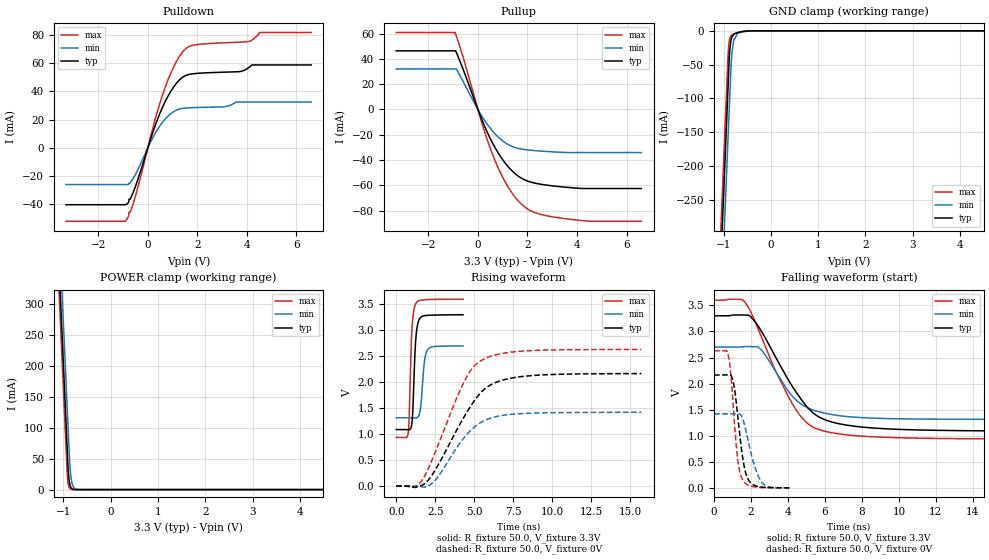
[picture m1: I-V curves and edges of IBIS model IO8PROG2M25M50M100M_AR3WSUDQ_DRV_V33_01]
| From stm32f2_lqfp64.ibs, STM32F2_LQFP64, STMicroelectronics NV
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| *** New cell (Generated with 5.14beta1 (Sep 20 2010 13:23:23))
[Model]   IO8PROG2M25M50M100M_AR3WSUDQ_DRV_V33_01
Model_type 3-state
Polarity   Non-Inverting
Enable   Active-Low
| CAP_THRESHOLD on pad IOV33 is "CMOS" :
| Rising=10.0% of vddio   Falling=90.0% of vddio
| C_comp min and max val. don't necessarily correlate with the min and max pvt
| but are the smallest and greatest pad capacitance found.
| var   typ   min   max
C_comp   2.51830pF  2.40455pF  2.66130pF
Vmeas = 1.65V   | Reference voltage for timing measurements
Cref  = 50.0pF   | Timing specification test load capacitance value
Rref  = 1.0MOhm   | Timing specification test load resistance value
Vref  = 1.65V   | Timing specification test load voltage
[Model Spec]
| variable   typ   min   max
[Temperature Range] 25.0 125.0 -40.0
| variable   typ   min   max
[Voltage Range] 3.3V 2.7V 3.6V
| variable   typ   min   max
[POWER Clamp Reference] 3.3V 2.7V 3.6V
| variable   typ   min   max
[GND Clamp Reference] 0V 0V 0V
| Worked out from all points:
|   slope of the pulldown table from 0 to 0.495 V, typ, clamps not added: 20 ohm
|   slope of the pullup table from 0 to 0.495 V, typ, clamps not added: 21.7 ohm
|   GND clamp passes 1 mA (typ) near -0.59 V on its own axis
|   POWER clamp passes 1 mA (typ) near -0.81 V on its own axis
|   rising waveform, R_fixture 50.0, V_fixture 3.3V: 20-80 % time 186ps typ, 225ps min, 175ps max; typ from 1.09 V to 3.3 V
|   falling waveform, R_fixture 50.0, V_fixture 3.3V: 20-80 % time 2.29ns typ, 1.78ns min, 2.13ns max; typ from 3.3 V to 1.09 V
|   rising waveform, R_fixture 50.0, V_fixture 0V: 20-80 % time 2.49ns typ, 2.08ns min, 2.18ns max; typ from 0 V to 2.17 V
|   falling waveform, R_fixture 50.0, V_fixture 0V: 20-80 % time 445ps typ, 627ps min, 360ps max; typ from 2.17 V to 0.001 V
[POWER Clamp]
-3.3V     4.117A     4.183A     4.076A
-1.09V    360mA      425.6mA    319.3mA
-1.05V    292mA      357.6mA    251.3mA
-1.01V    224mA      289.6mA    183.3mA
-910mV    53.96mA    119.6mA    18.43mA
-900mV    36.96mA    102.6mA    11.2mA
-880mV    16.97mA    68.61mA    4.141mA
-860mV    7.791mA    38.56mA    1.53mA
-840mV    3.577mA    21.53mA    565.5uA
-780mV    346.2uA    3.745mA    28.55uA
-660mV    3.242uA    113.2uA    73.21nA
6.6V      0A         0A         0A
[GND Clamp]
-3.3V     -4.156A    -4.231A    -4.108A
-1.06V    -347.5mA   -423.2mA   -300.1mA
-940mV    -143.5mA   -219.2mA   -96.09mA
-900mV    -75.54mA   -151.2mA   -30.39mA
-880mV    -41.78mA   -117.2mA   -15.62mA
-870mV    -30.28mA   -100.2mA   -12.04mA
-840mV    -13.1mA    -50.87mA   -7.186mA
-820mV    -8.54mA    -30.65mA   -5.881mA
-780mV    -4.86mA    -12.37mA   -4.416mA
-700mV    -2.552mA   -3.603mA   -2.454mA
-350mV    -11.93uA   -60.06uA   -2.46uA
6.6V      10.25nA    1.32uA     122.8pA
| variable   typ   min   max
[Pullup Reference] 3.3V 2.7V 3.6V
| variable   typ   min   max
[Pulldown Reference] 0V 0V 0V
[Pullup]
-3.3V     46.44mA    32.07mA    60.89mA
-920mV    46.44mA    32.07mA    60.89mA
-870mV    45.09mA    32.07mA    58.1mA
-590mV    31.41mA    21.87mA    40.86mA
240mV     -11.89mA   -7.822mA   -15.87mA
590mV     -26.5mA    -17.07mA   -35.52mA
1.18V     -44.36mA   -27.27mA   -60.11mA
1.54V     -51.43mA   -30.39mA   -70.35mA
1.89V     -55.75mA   -31.69mA   -77.18mA
2.48V     -58.98mA   -32.83mA   -82.75mA
3.6V      -61.62mA   -34.07mA   -86.61mA
6.6V      -62.54mA   -34.07mA   -88.51mA
[Pulldown]
-3.3V     -40.26mA   -25.94mA   -51.99mA
-910mV    -40.26mA   -25.94mA   -51.99mA
-820mV    -39.59mA   -25.94mA   -49.78mA
-470mV    -25.89mA   -17.87mA   -32.39mA
240mV     12.97mA    8.52mA     16.62mA
590mV     28.62mA    18.11mA    37.2mA
1.07V     43.85mA    26mA       58.31mA
1.54V     51.42mA    28.24mA    70.48mA
2.01V     52.82mA    28.63mA    73.27mA
4.01V     56.04mA    32.48mA    75.18mA
4.52V     58.77mA    32.48mA    81.71mA
6.6V      58.77mA    32.48mA    81.71mA
[Ramp]
dV/dt_r 1.29886V/2.48883ns 851.30655mV/2.08394ns 1.57727V/2.18373ns
dV/dt_f 1.32782V/2.29052ns 831.60246mV/1.77805ns 1.59819V/2.12819ns
R_load = 50.0
| Removed startup time: 0s 0s 0s  .
| Removed end time: 4.279ns.
[Rising Waveform]
R_fixture   = 50.0
V_fixture   = 3.3V
V_fixture_min = 2.7V
V_fixture_max = 3.6V
0s        1.087V     1.314V     936.3mV
766ps     1.084V     1.314V     1.014V
820ps     1.083V     1.314V     1.252V
938ps     1.116V     1.314V     2.555V
1.027ns   1.267V     1.313V     3.108V
1.242ns   2.778V     1.309V     3.51V
1.537ns   3.239V     1.457V     3.577V
1.802ns   3.279V     2.384V     3.586V
2.006ns   3.286V     2.622V     3.589V
4.281ns   3.298V     2.698V     3.598V
| Removed startup time: 0s 0s 0s  .
| Removed end time: 20.2ns.
[Falling Waveform]
R_fixture   = 50.0
V_fixture   = 3.3V
V_fixture_min = 2.7V
V_fixture_max = 3.6V
0s        3.3V       2.7V       3.6V
1.655ns   3.316V     2.711V     3.568V
1.975ns   3.285V     2.711V     3.382V
2.52ns    3.03V      2.66V      2.931V
4.19ns    1.969V     1.778V     1.642V
4.915ns   1.602V     1.562V     1.283V
5.595ns   1.378V     1.467V     1.128V
6.84ns    1.224V     1.382V     1.032V
9.205ns   1.135V     1.331V     970.7mV
20.21ns   1.087V     1.314V     936.6mV
| Removed startup time: 0s 0s 0s  .
| Removed end time: 15.69ns.
[Rising Waveform]
R_fixture   = 50.0
V_fixture   = 0V
V_fixture_min = 0V
V_fixture_max = 0V
0s        8.532nV    394.5nV    5.735nV
920ps     -7.581mV   78.62uV    -35.54mV
1.67ns    16.63mV    -16.62mV   117.4mV
2.535ns   325.7mV    122.6mV    676mV
4.395ns   1.357V     949.1mV    2.036V
4.89ns    1.592V     1.105V     2.274V
5.47ns    1.814V     1.232V     2.422V
6.415ns   2V         1.338V     2.529V
7.975ns   2.106V     1.394V     2.596V
15.7ns    2.165V     1.419V     2.629V
| Removed startup time: 0s 0s 0s  .
| Removed end time: 4.064ns.
[Falling Waveform]
R_fixture   = 50.0
V_fixture   = 0V
V_fixture_min = 0V
V_fixture_max = 0V
0s        2.165V     1.419V     2.629V
773ps     2.17V      1.418V     2.542V
882ps     2.165V     1.418V     2.266V
1.029ns   2.043V     1.42V      1.6V
1.258ns   1.443V     1.426V     605.4mV
1.536ns   607.6mV    1.339V     160.3mV
1.885ns   138.5mV    837.2mV    44.76mV
2.23ns    42.42mV    378.2mV    17.62mV
2.566ns   14.96mV    114.4mV    7.159mV
4.066ns   1.242mV    1.365mV    949uV
